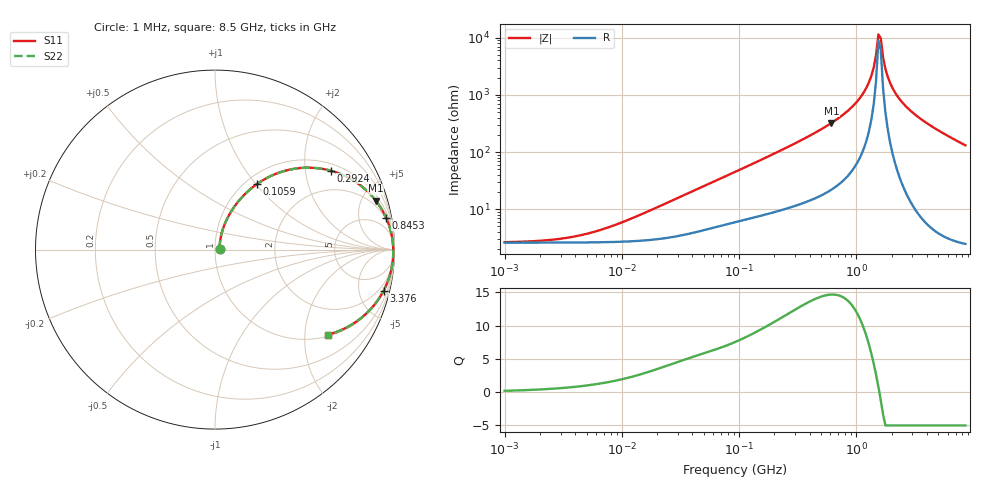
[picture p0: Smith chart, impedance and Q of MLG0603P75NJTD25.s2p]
! S-Parameter Data Generated by TDK Corporation
! Copyright(C) 2025 TDK Corporation.
! All Rights Reserved.
! TDK P/N: MLG0603P75NJTD25 (SMD / SMT Inductor (Coil))
! Property: L=75nH at 300MHz
! Size(LxWxT): 0.6x0.3x0.3mm
! Model Type: s2p (Touchstone File Format Version 1.0)
! Frequency: DC=Yes Start=1MHz Stop=8500MHz 198points Log-sweep
! Model Generated on Feb. 6, 2025
! Terms and conditions regarding TDK Simulation Models:
! 1)This simulation model is being provided solely for informational
!  purposes. Please refer to the specifications of the products in
!  terms of detailed characteristics of such products.
! 2)In no event shall TDK Corporation of any of its subsidiaries be
!  liable for any loss or damage arising, directly or indirectly,
!  from any information contained in this simulation model, including,
!  but not limited to loss or damages arising from any inaccuracies,
!  omissions or errors in connection with such information.
! 3)Any and all copyrights on this simulation model are owned by
!  TDK Corporation.  Duplication or redistribution of this simulation
!  model without prior written permission from TDK Corporation
!  is prohibited.
! 4)This simulation model is subject to any modification or change
!  without any prior notice.
! 5)Neither TDK Corporation nor any of its subsidiaries shall make any
!  warranty, express or implied, including but not limited to the
!  correctness, implied warranties of merchantability and fitness for
!  a particular purpose with respect to this simulation models.
! 6)The use of this simulation model shall be deemed to have consented
!  to the terms and conditions hereof.
! Port Assignments:
!  1 ---@@@--- 2
! Applicable Conditions:
!  Temperature = 25 degC
!  DC Bias Current = 0 A
!  Small Signal Operation
# Hz S MA R 50
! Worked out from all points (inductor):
!   197 points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, 1 MHz to 8.5 GHz, reference 50 ohm
!   read as one part in series: L = 82.3 nH near 16.71 MHz
!   highest Q = 14.7 at 611.9 MHz (marker M1), where L = 83.4 nH
!   self-resonance near 1.54 GHz
!   S11 on the Smith chart (normalised r, x): 1 MHz: 1.05, +0.01; 105.9 MHz: 1.13, +1.01; 292.4 MHz: 1.22, +2.75; 845.3 MHz: 2, +10; 3.376 GHz: 1.16, -8.13; 8.5 GHz: 1.05, -2.61
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1000000  0.02576 11.1  0.9747 -0.3  0.9747 -0.3  0.02576 11.1
4587603  0.03456 41.2  0.9743 -1.3  0.9743 -1.3  0.03456 41.2
2.10461e7  0.109 68.5  0.9653 -6.0  0.9653 -6.0  0.109 68.5
9.219544e7  0.3901 59.7  0.8708 -22.7  0.8708 -22.7  0.3901 59.7
1.058897e8  0.4333 57.4  0.8491 -25.5  0.8491 -25.5  0.4333 57.4
1.842597e8  0.6263 45.8  0.7209 -38.6  0.7209 -38.6  0.6263 45.8
2.923552e8  0.7804 34.3  0.5652 -51.1  0.5652 -51.1  0.7804 34.3
4.229561e8  0.8745 25.1  0.426 -60.7  0.426 -60.7  0.8745 25.1
6.11899e8  0.937 16.9  0.2915 -69.2  0.2915 -69.2  0.937 16.9
8.453103e8  0.9696 10.6  0.1842 -75.3  0.1842 -75.3  0.9696 10.6
1.064771e9  0.9834 6.5  0.1134 -78.4  0.1134 -78.4  0.9834 6.5
1.280704e9  0.99 3.4  0.05929 -78.6  0.05929 -78.6  0.99 3.4
1.404574e9  0.992 1.8  0.03289 -75.0  0.03289 -75.0  0.992 1.8
1.470933e9  0.9927 1.1  0.02005 -68.1  0.02005 -68.1  0.9927 1.1
1.540426e9  0.9932 0.3  0.00872 -38.3  0.00872 -38.3  0.9932 0.3
1.613203e9  0.9934 -0.5  0.01021 49.9  0.01021 49.9  0.9934 -0.5
1.689417e9  0.9935 -1.2  0.0221 72.3  0.0221 72.3  0.9935 -1.2
1.769233e9  0.9934 -2.0  0.03511 78.2  0.03511 78.2  0.9934 -2.0
1.940355e9  0.9925 -3.5  0.06186 81.3  0.06186 81.3  0.9925 -3.5
2.444114e9  0.9864 -7.5  0.1315 80.3  0.1315 80.3  0.9864 -7.5
3.37643e9  0.9665 -13.8  0.2378 75.1  0.2378 75.1  0.9665 -13.8
8.5e9  0.7872 -37.0  0.602 51.9  0.602 51.9  0.7872 -37.0
